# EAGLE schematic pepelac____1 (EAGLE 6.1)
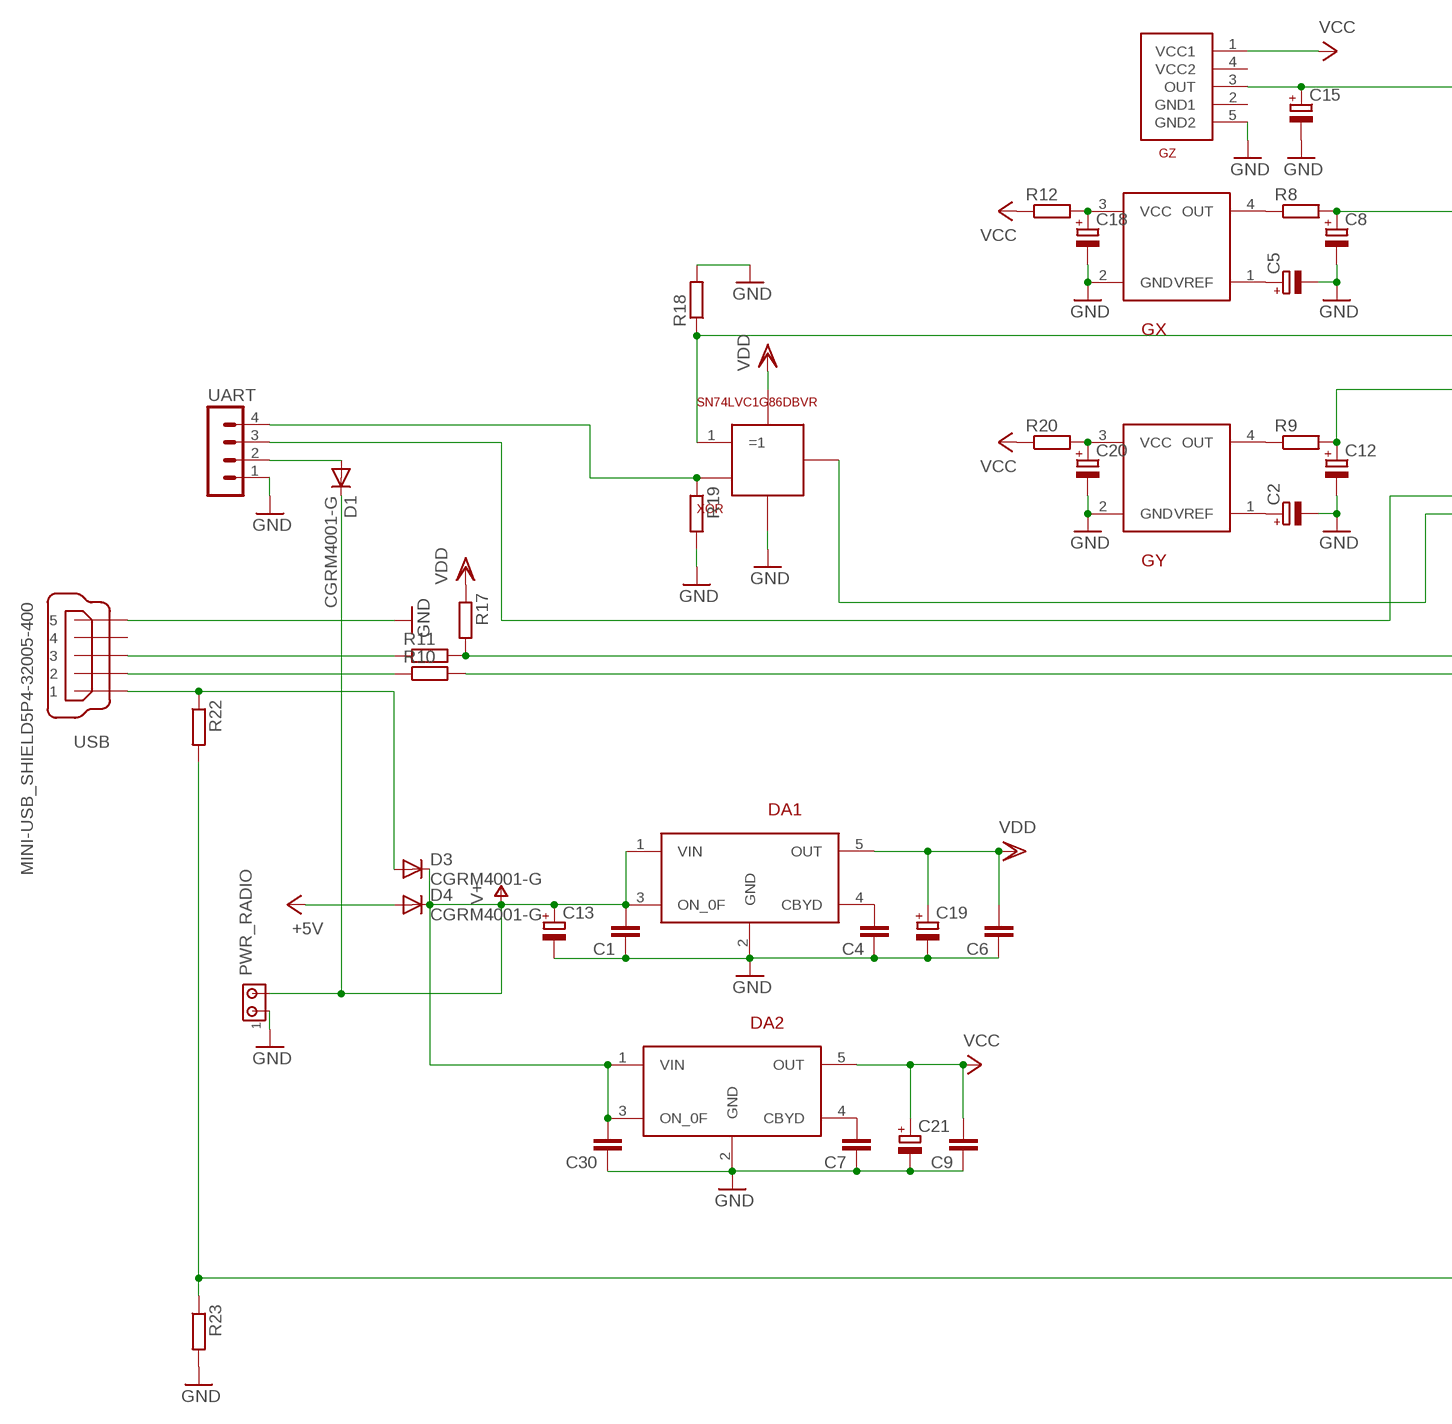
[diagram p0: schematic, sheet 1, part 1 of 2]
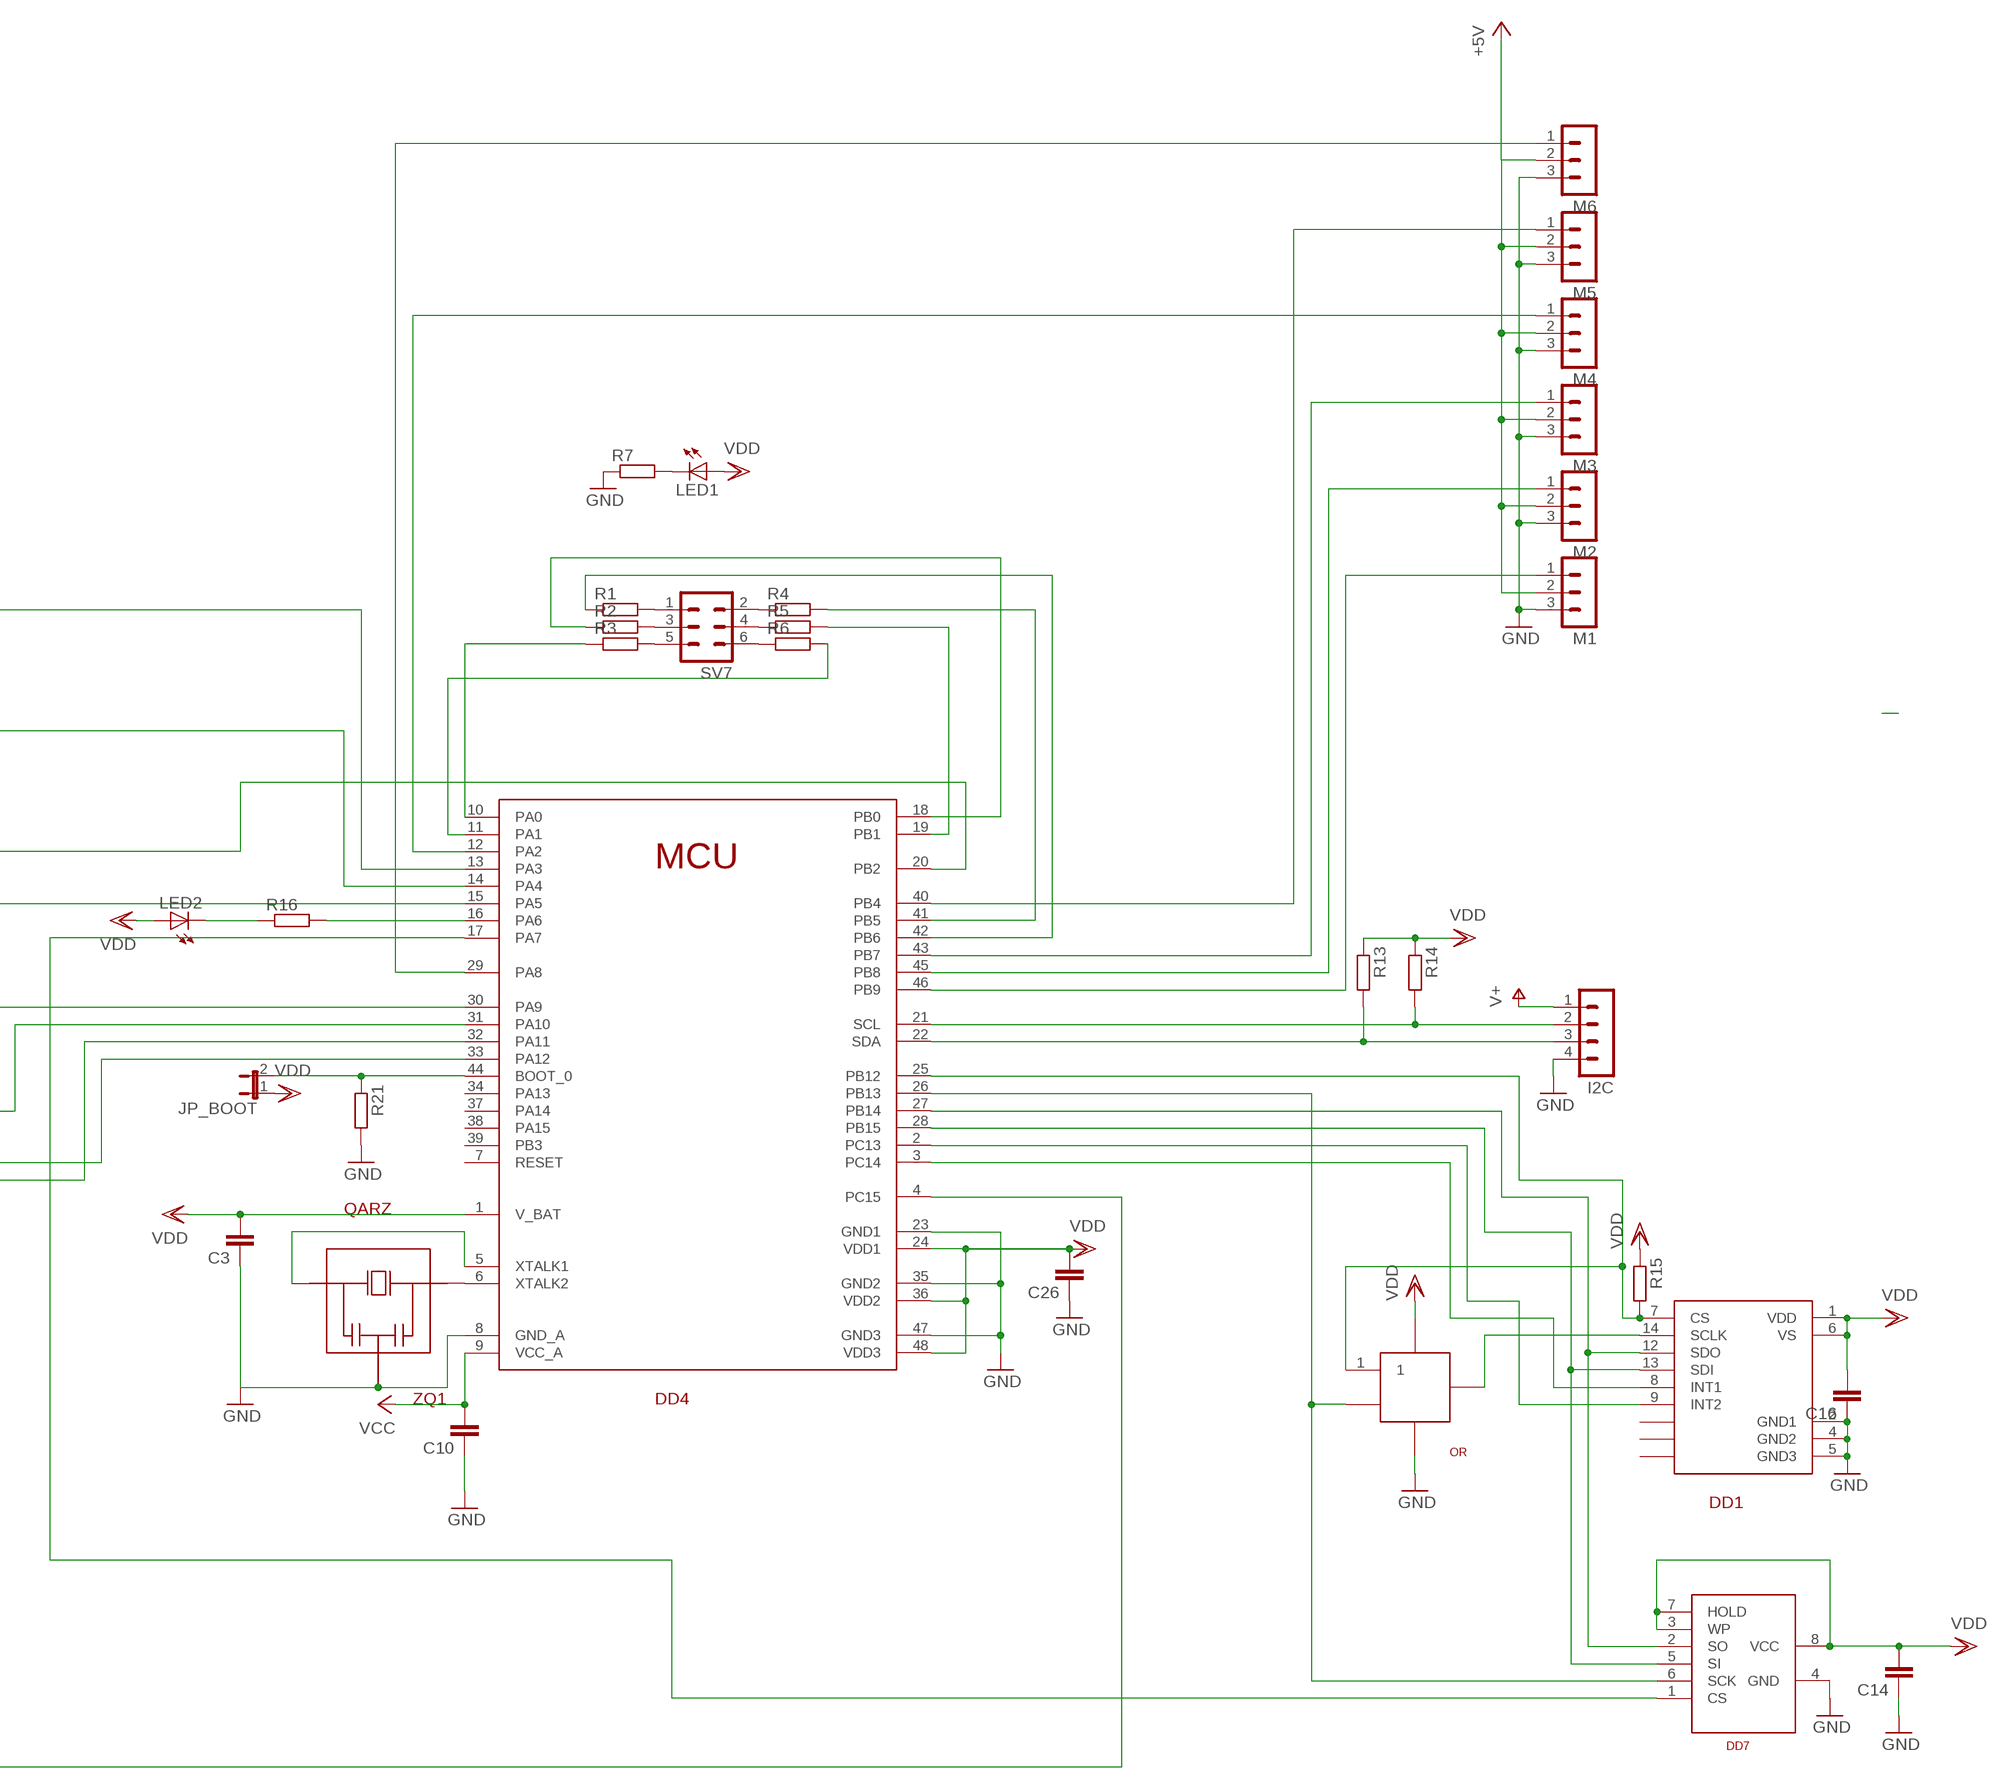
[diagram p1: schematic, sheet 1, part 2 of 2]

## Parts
C1  C-EUC0603K  [C0603K]
C2  CPOL-EUB/3528-21R  [B/3528-21R]
C3  C-EUC0603K  [C0603K]
C4  C-EUC0603K  [C0603K]
C5  CPOL-EUB/3528-21R  [B/3528-21R]
C6  C-EUC0603K  [C0603K]
C7  C-EUC0603K  [C0603K]
C8  CPOL-EUB/3528-21R  [B/3528-21R]
C9  C-EUC0603K  [C0603K]
C10  C-EUC0603K  [C0603K]
C12  CPOL-EUB/3528-21R  [B/3528-21R]
C13  CPOL-EUB/3528-21R  [B/3528-21R]
C14  C-EUC0603K  [C0603K]
C15  CPOL-EUB/3528-21R  [B/3528-21R]
C16  C-EUC0603K  [C0603K]
C18  CPOL-EUB/3528-21R  [B/3528-21R]
C19  CPOL-EUB/3528-21R  [B/3528-21R]
C20  CPOL-EUB/3528-21R  [B/3528-21R]
C21  CPOL-EUB/3528-21R  [B/3528-21R]
C26  C-EUC0603K  [C0603K]
C30  C-EUC0603K  [C0603K]
D1  CGRM4001-G  [SOD-123_MINI-SMA]
D3  CGRM4001-G  [SOD-123_MINI-SMA]
D4  CGRM4001-G  [SOD-123_MINI-SMA]
DA1  3.3  [SC70-5L]
DA2  3.3  [SC70-5L]
DD1  ADXL345  [ACC]
DD4  PROC  [LQFP48]
DD7  W25X40  [SOIC8]
GX  GIROSCOPE  [GIRO]
GY  GIROSCOPE  [GIRO]
GZ  GZ-03  [GZ]
I2C  MA04-1  [MA04-1]
JP_BOOT  JP1E  [JP1]
LED1  LEDCHIP-LED0603  [CHIP-LED0603]
LED2  LEDCHIP-LED0603  [CHIP-LED0603]
M1  MA03-1  [MA03-1]
M2  MA03-1  [MA03-1]
M3  MA03-1  [MA03-1]
M4  MA03-1  [MA03-1]
M5  MA03-1  [MA03-1]
M6  MA03-1  [MA03-1]
OR  SN74AHC1G32  [SOT23-5L]
PWR_RADIO  MTA02-100  [10X02MTA]
R1  R-EU_MELF0102W  [MINI_MELF-0102W]
R2  R-EU_MELF0102W  [MINI_MELF-0102W]
R3  R-EU_MELF0102W  [MINI_MELF-0102W]
R4  R-EU_MELF0102W  [MINI_MELF-0102W]
R5  R-EU_MELF0102W  [MINI_MELF-0102W]
R6  R-EU_MELF0102W  [MINI_MELF-0102W]
R7  R-EU_MELF0102W  [MINI_MELF-0102W]
R8  R-EU_MELF0102W  [MINI_MELF-0102W]
R9  R-EU_MELF0102W  [MINI_MELF-0102W]
R10  R-EU_MELF0102W  [MINI_MELF-0102W]
R11  R-EU_MELF0102W  [MINI_MELF-0102W]
R12  R-EU_MELF0102W  [MINI_MELF-0102W]
R13  R-EU_MELF0102W  [MINI_MELF-0102W]
R14  R-EU_MELF0102W  [MINI_MELF-0102W]
R15  R-EU_MELF0102W  [MINI_MELF-0102W]
R16  R-EU_MELF0102W  [MINI_MELF-0102W]
R17  R-EU_MELF0102W  [MINI_MELF-0102W]
R18  R-EU_MELF0102W  [MINI_MELF-0102W]
R19  R-EU_MELF0102W  [MINI_MELF-0102W]
R20  R-EU_MELF0102W  [MINI_MELF-0102W]
R21  R-EU_MELF0102W  [MINI_MELF-0102W]
R22  R-EU_MELF0102W  [MINI_MELF-0102W]
R23  R-EU_MELF0102W  [MINI_MELF-0102W]
SV7  MA03-2  [MA03-2]
UART  MA04-1  [MA04-1]
USB  MINI-USB_SHIELD5P4-32005-400  [32005-400]
XOR  SN74LVC1G86DBVR  [SOT23-5L]
ZQ1  QARZ  [QARZ]

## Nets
+5V: D4.A M1.2 M2.2 M3.2 M4.2 M5.2 M6.2
GND: C1.1 C2.- C3.1 C4.1 C5.- C6.1 C7.1 C8.- C9.1 C10.1 C12.- C13.- C14.1 C15.- C16.1 C18.- C19.- C20.- C21.- C26.1 C30.1 DA1.2(GND) DA2.2(GND) DD1.2(GND1) DD1.4(GND2) DD1.5(GND3) DD4.8(GND_A) DD4.23(GND1) DD4.35(GND2) DD4.47(GND3) DD7.4(GND) GX.2(GND) GY.2(GND) GZ.5(GND2) I2C.4 M1.3 M2.3 M3.3 M4.3 M5.3 M6.3 OR.3 PWR_RADIO.1 R7.1 R18.2 R19.2 R21.2 R23.2 UART.1 USB.5 XOR.3 ZQ1.2
N$1: DD4.6(XTALK2) ZQ1.3
N$2: GX.4(OUT) R8.1
N$3: GY.4(OUT) R9.1
N$4: DD1.7(CS) DD4.25(PB12) OR.1 R15.2
N$5: DD4.16(PA6) R16.2
N$6: DD4.33(PA12) R11.2 R17.2
N$7: DD4.29(PA8) M6.1
N$8: D1.A UART.2
N$9: C18.+ GX.3(VCC) R12.2
N$10: C20.+ GY.3(VCC) R20.2
N$11: DD1.9(INT2) DD4.2(PC13)
N$12: LED2.C R16.1
N$13: C7.2 DA2.4(CBYD)
N$14: C12.+ DD4.15(PA5) R9.2
N$15: C8.+ DD4.14(PA4) R8.2
N$16: LED1.C R7.2
N$17: DD1.8(INT1) DD4.3(PC14)
N$18: C2.+ GY.1(VREF)
N$19: R1.2 SV7.1
N$20: R2.2 SV7.3
N$21: R3.2 SV7.5
N$22: R4.1 SV7.2
N$23: R5.1 SV7.4
N$24: R6.1 SV7.6
N$25: DD4.42(PB6) R1.1
N$26: DD4.41(PB5) R4.2
N$27: DD4.18(PB0) R2.1
N$28: DD4.19(PB1) R5.2
N$29: DD4.10(PA0) R3.1
N$30: DD4.11(PA1) R6.2
N$31: C15.+ DD4.13(PA3) GZ.3(OUT)
N$32: DD4.5(XTALK1) ZQ1.1
N$34: DD4.46(PB9) M1.1
N$35: DD4.45(PB8) M2.1
N$36: DD4.43(PB7) M3.1
N$37: DD4.40(PB4) M5.1
N$38: DD4.12(PA2) M4.1
N$39: C5.+ GX.1(VREF)
N$40: R19.1 UART.4 XOR.2
N$41: C4.2 DA1.4(CBYD)
N$43: DD4.30(PA9) UART.3
N$44: DD4.4(PC15) R22.2 R23.1
N$45: D3.A R22.1 USB.1
N$46: R10.1 USB.2
N$47: R11.1 USB.3
N$48: DD4.20(PB2) R18.1 XOR.1(=1)
N$49: DD4.31(PA10) XOR.4
N$50: DD4.22(SDA) I2C.3 R13.2
N$51: DD4.21(SCL) I2C.2 R14.2
N$53: DD4.32(PA11) R10.2
N$54: DD4.44(BOOT_0) JP_BOOT.2 R21.1
N$58: DD4.17(PA7) DD7.1(CS)
N$60: DD4.26(PB13) DD7.6(SCK) OR.2
N$61: DD1.12(SDO) DD4.27(PB14) DD7.2(SO)
N$62: DD1.14(SCLK) OR.5
N$63: DD1.13(SDI) DD4.28(PB15) DD7.5(SI)
V+: C1.2 C13.+ C30.2 D1.C D3.C D4.C DA1.1(VIN) DA1.3(ON_0F) DA2.1(VIN) DA2.3(ON_0F) I2C.1 PWR_RADIO.2
VCC: C9.2 C10.2 C21.+ DA2.5(OUT) DD4.9(VCC_A) GZ.1(VCC1) R12.1 R20.1
VDD: C3.2 C6.2 C14.2 C16.2 C19.+ C26.2 DA1.5(OUT) DD1.1(VDD) DD1.6(VS) DD4.1(V_BAT) DD4.24(VDD1) DD4.36(VDD2) DD4.48(VDD3) DD7.3(WP) DD7.7(HOLD) DD7.8(VCC) JP_BOOT.1 LED1.A LED2.A OR.4 R13.1 R14.1 R15.1 R17.1 XOR.5
Unconnected: DD1.3 DD1.10 DD1.11 DD4.7(RESET) DD4.34(PA13) DD4.37(PA14) DD4.38(PA15) DD4.39(PB3) GZ.2(GND1) GZ.4(VCC2) USB.4 USB.M1(S1) USB.M2(S2) USB.M3(S3) USB.M4(S4)

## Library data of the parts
C1 C3 C4 C6 C7 C9 C10 C14 C16 C26 C30 = resistor:C-EU: CAPACITOR, European symbol
C2 C5 C8 C12 C13 C15 C18-C21 = rcl:CPOL-EU: POLARIZED CAPACITOR, European symbol
D1 D3 D4 = diode:CGRM400*-G: Molded plasitc,JEDEC SOD-123/Mini SMA
DA1 DA2 = pepelac:3.3
DD1 = pepelac:ADXL345
DD4 = pepelac:PROC
DD7 = pepelac:W25X40
GX GY = pepelac:GIROSCOPE
GZ = pepelac:GZ-03
I2C UART = con-lstb:MA04-1: PIN HEADER; OC_FARNELL: unknown; OC_NEWARK: unknown
JP_BOOT = jumper:JP1E: JUMPER
LED1 LED2 = led:LED: LED
M1-M6 = con-lstb:MA03-1: PIN HEADER; OC_FARNELL: unknown; OC_NEWARK: unknown
OR = pepelac:SN74AHC1G32
PWR_RADIO = con-amp:MTA02-100: AMP connector
R1-R23 = resistor:R-EU_: RESISTOR, European symbol
SV7 = con-lstb:MA03-2: PIN HEADER; OC_FARNELL: unknown; OC_NEWARK: unknown
USB = con-cypressindustries:MINI-USB_SHIELD5P4-: MINI USB-B R/A W/O POST 5 pol. Source: www.cypressindustries.com; OC_FARNELL: unknown; OC_NEWARK: unknown
XOR = pepelac:SN74LVC1G86DBVR
ZQ1 = pepelac:QARZ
